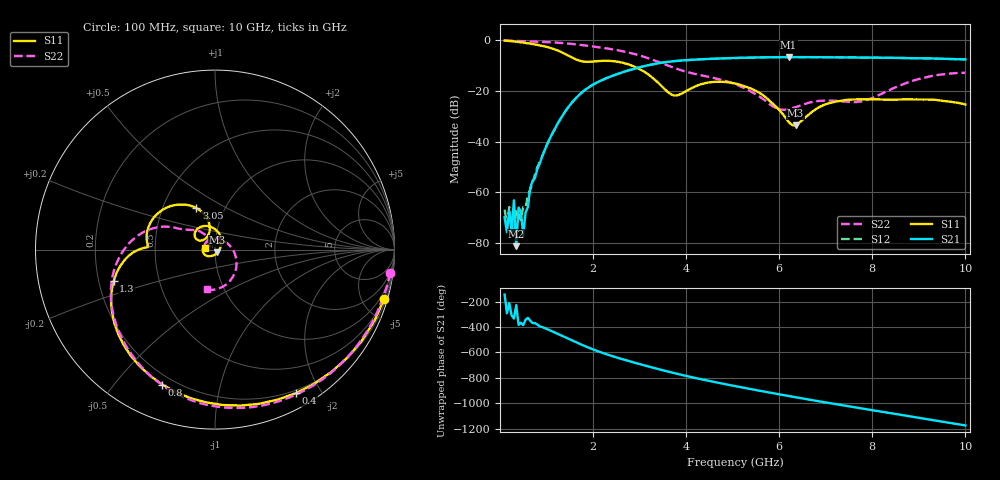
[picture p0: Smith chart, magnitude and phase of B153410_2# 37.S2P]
!  2-Port S-parameters saved by WinCal
! VAR MeasName=S-Parameters (CALIBRATED_DATA) read from VNA (N5245A)
! VAR MeasDate=2016-12-23 10:01:15
! VAR NAME=B153410_2# 37
! VAR FILENAME=B153410_2# 37.S2P
! VAR DATE=2016-12-23 10:01:15
! VAR PHYS_PORTS=1,2
# Hz S DB R 50
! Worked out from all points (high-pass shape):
!   199 points, 100 MHz to 10 GHz, reference 50 ohm
!   highest |S21| = -6.69 dB at 6.2 GHz (marker M1); lowest = -81.2 dB at 350 MHz (marker M2)
!   |S21| within 3 dB of the highest: 3.238 GHz to end of sweep
!   lowest |S11| = -33.7 dB at 6.35 GHz (marker M3), VSWR 1.04, Z = 51.4 - j1.59 ohm
!   |S11| at or under -10 dB: 2.826 GHz to end of sweep
!   |S22| runs from -27.5 to -0.1 dB; largest |S21 - S12| = 0.0023
!   S11 on the Smith chart (normalised r, x): 100 MHz: 0.46, -7.03; 400 MHz: 0.17, -1.70; 800 MHz: 0.16, -0.67; 1.3 GHz: 0.26, -0.14; 3.05 GHz: 0.74, +0.36; 10 GHz: 0.90, +0.02
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1e8  -0.16 -16.1  -69.86 -144.4  -66.81 105.8  -0.13 -7.5
1.5e8  -0.24 -23.9  -75.75 68.2  -72.65 23.3  -0.17 -11.0
2e8  -0.33 -31.5  -67.24 148.1  -65.80 22.4  -0.21 -14.4
2.5e8  -0.42 -39.0  -75.18 52.5  -74.69 -52.5  -0.25 -17.6
3e8  -0.53 -46.2  -63.16 27.0  -76.38 -103.6  -0.28 -21.0
3.5e8  -0.63 -53.4  -81.24 132.5  -66.95 3.8  -0.31 -24.3
4e8  -0.74 -60.5  -66.01 -23.3  -68.65 6.0  -0.33 -27.6
5e8  -0.98 -74.1  -76.91 -25.1  -65.81 49.3  -0.39 -34.2
6.5e8  -1.38 -93.4  -58.36 10.6  -58.85 0.1  -0.48 -44.1
8e8  -1.86 -111.3  -51.02 -19.4  -50.19 -20.6  -0.59 -53.9
1.3e9  -4.55 -162.7  -31.09 -103.5  -31.03 -103.0  -1.09 -86.0
1.75e9  -8.31 178.2  -20.81 -178.2  -20.78 -178.1  -1.92 -113.7
3.05e9  -11.91 114.2  -10.47 23.5  -10.46 23.5  -6.32 176.2
3.4e9  -16.81 102.4  -9.14 -10.8  -9.13 -10.7  -8.57 161.9
3.75e9  -21.84 128.2  -8.28 -43.2  -8.26 -43.1  -11.00 153.4
4.25e9  -17.85 148.9  -7.61 -85.2  -7.61 -85.2  -13.58 147.6
5.05e9  -17.11 109.4  -7.04 -144.8  -7.05 -144.8  -17.31 130.8
6.2e9  -32.22 0.2  -6.69 137.2  -6.70 137.4  -27.24 158.7
6.35e9  -33.65 -48.1  -6.69 127.5  -6.70 127.6  -26.43 166.0
6.7e9  -28.35 -115.0  -6.71 105.3  -6.70 105.3  -24.43 163.3
8.35e9  -23.49 -174.7  -6.97 4.6  -6.95 4.6  -19.82 -2.5
1e10  -25.39 170.2  -7.61 -94.4  -7.65 -94.3  -12.90 -101.7
